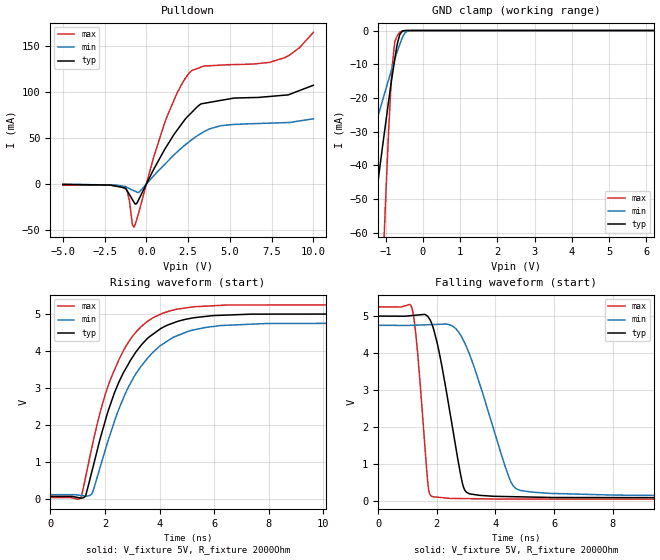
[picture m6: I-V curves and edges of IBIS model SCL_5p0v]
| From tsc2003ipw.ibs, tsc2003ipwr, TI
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|   SCL_5p0v
[Model]   SCL_5p0v
Model_type   I/O_open_drain
Polarity   Non-Inverting
Enable   Active-High
Vinl = 1.5
Vinh = 3.5
Vmeas = 2.5
Vref = 2.5
Cref = 1pF
Rref = 50
|   typ   min   max
C_comp   0.464pF   0.356pF   0.523pF
[Voltage Range]   5   4.75   5.25
[Temperature Range]   27   85   -40
[Pullup Reference]   5   4.75   5.25
[Pulldown Reference]   0   0   0
[Power Clamp Reference]   5   4.75   5.25
[GND Clamp Reference]   0   0   0
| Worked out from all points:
|   slope of the pulldown table from 0 to 0.75 V, typ, clamps not added: 28.7 ohm
|   GND clamp passes 1 mA (typ) near -0.60 V on its own axis
|   falling waveform, V_fixture 5V, R_fixture 2000Ohm: 20-80 % time 650ps typ, 1.1ns min, 310ps max; typ from 5 V to 0.065 V
|   rising waveform, V_fixture 5V, R_fixture 2000Ohm: 20-80 % time 1.55ns typ, 1.69ns min, 1.41ns max; typ from 0.064 V to 5 V
[Pulldown]
|   Voltage   I(typ)   I(min)   I(max)
-5V       -323uA     -235.9uA   -1.276mA
-1.235V   -4.526mA   -2.718mA   -5.152mA
-1.01V    -11.4mA    -5.001mA   -18.19mA
-832.6mV  -16.81mA   -6.508mA   -44.3mA
-737.2mV  -19.72mA   -7.245mA   -46.69mA
-543.3mV  -19.95mA   -8.743mA   -36.35mA
1.06V     36.37mA    20.66mA    64.27mA
2.595V    75.47mA    46.35mA    121mA
3.278V    86.95mA    54.83mA    126.8mA
4.429V    90.6mA     63.15mA    128.9mA
8.265V    96.32mA    66.56mA    136.9mA
10V       107.1mA    70.76mA    164.5mA
[GND Clamp]
|   Voltage   I(typ)   I(min)   I(max)
-5V       -381.2mA   -176.9mA   -1.217A
-2.135V   -126.2mA   -62.06mA   -376.8mA
-1.535V   -73.45mA   -38.34mA   -201.6mA
-1.246V   -48.43mA   -27.06mA   -118.6mA
-1.076V   -33.97mA   -20.55mA   -71.34mA
-1.01V    -28.52mA   -18.03mA   -53.24mA
-919.2mV  -21.06mA   -14.63mA   -30.13mA
-832.6mV  -14.21mA   -11.47mA   -11.7mA
-755.7mV  -8.746mA   -8.666mA   -3.631mA
-552.6mV  -264.5uA   -2.19mA    -112.3uA
-301.4mV  -835.7nA   -5.809uA   -4.318uA
10V       0A         0A         0A
[POWER Clamp]
|   Voltage   I(typ)   I(min)   I(max)
-5V       0A         0A         0A
0V        0A         0A         0A
10V       0A         0A         0A
[Ramp]
R_load = 2000
|   typ   min   max
dV/dt_r   2.96158/1.55284e-009   2.78437/1.69065e-009   3.12914/1.40821e-009
dV/dt_f   2.96103/6.49734e-010   2.7813/1.10025e-009   3.12913/3.08829e-010
[Falling Waveform]
V_fixture = 5V
V_fixture_min = 4.75V
V_fixture_max = 5.25V
R_fixture = 2000Ohm
C_fixture = 0F
|   Time   V(typ)   V(min)   V(max)
0s        5V         4.75V      5.25V
1.154ns   5.015V     4.75V      5.211V
1.339ns   5.029V     4.755V     4.067V
1.699ns   4.986V     4.766V     443.5mV
1.858ns   4.73V      4.771V     106.3mV
2.86ns    519.3mV    4.418V     55.64mV
3.118ns   184.4mV    3.96V      52.87mV
4.49ns    107.9mV    574.6mV    41.96mV
4.849ns   102.2mV    276.9mV    41.8mV
20.94ns   64.94mV    114.5mV    34.78mV
[Rising Waveform]
V_fixture = 5V
V_fixture_min = 4.75V
V_fixture_max = 5.25V
R_fixture = 2000Ohm
C_fixture = 0F
|   Time   V(typ)   V(min)   V(max)
0s        64.02mV    109.4mV    34.76mV
1.124ns   17.16mV    87mV       20.59mV
1.28ns    61.64mV    70.53mV    536.6mV
1.504ns   677.5mV    116.3mV    1.32V
2.01ns    2.099V     1.31V      2.811V
2.689ns   3.42V      2.739V     4.017V
3.314ns   4.137V     3.57V      4.639V
4.123ns   4.632V     4.182V     5.015V
6.237ns   4.958V     4.681V     5.227V
20.94ns   5V         4.75V      5.25V
